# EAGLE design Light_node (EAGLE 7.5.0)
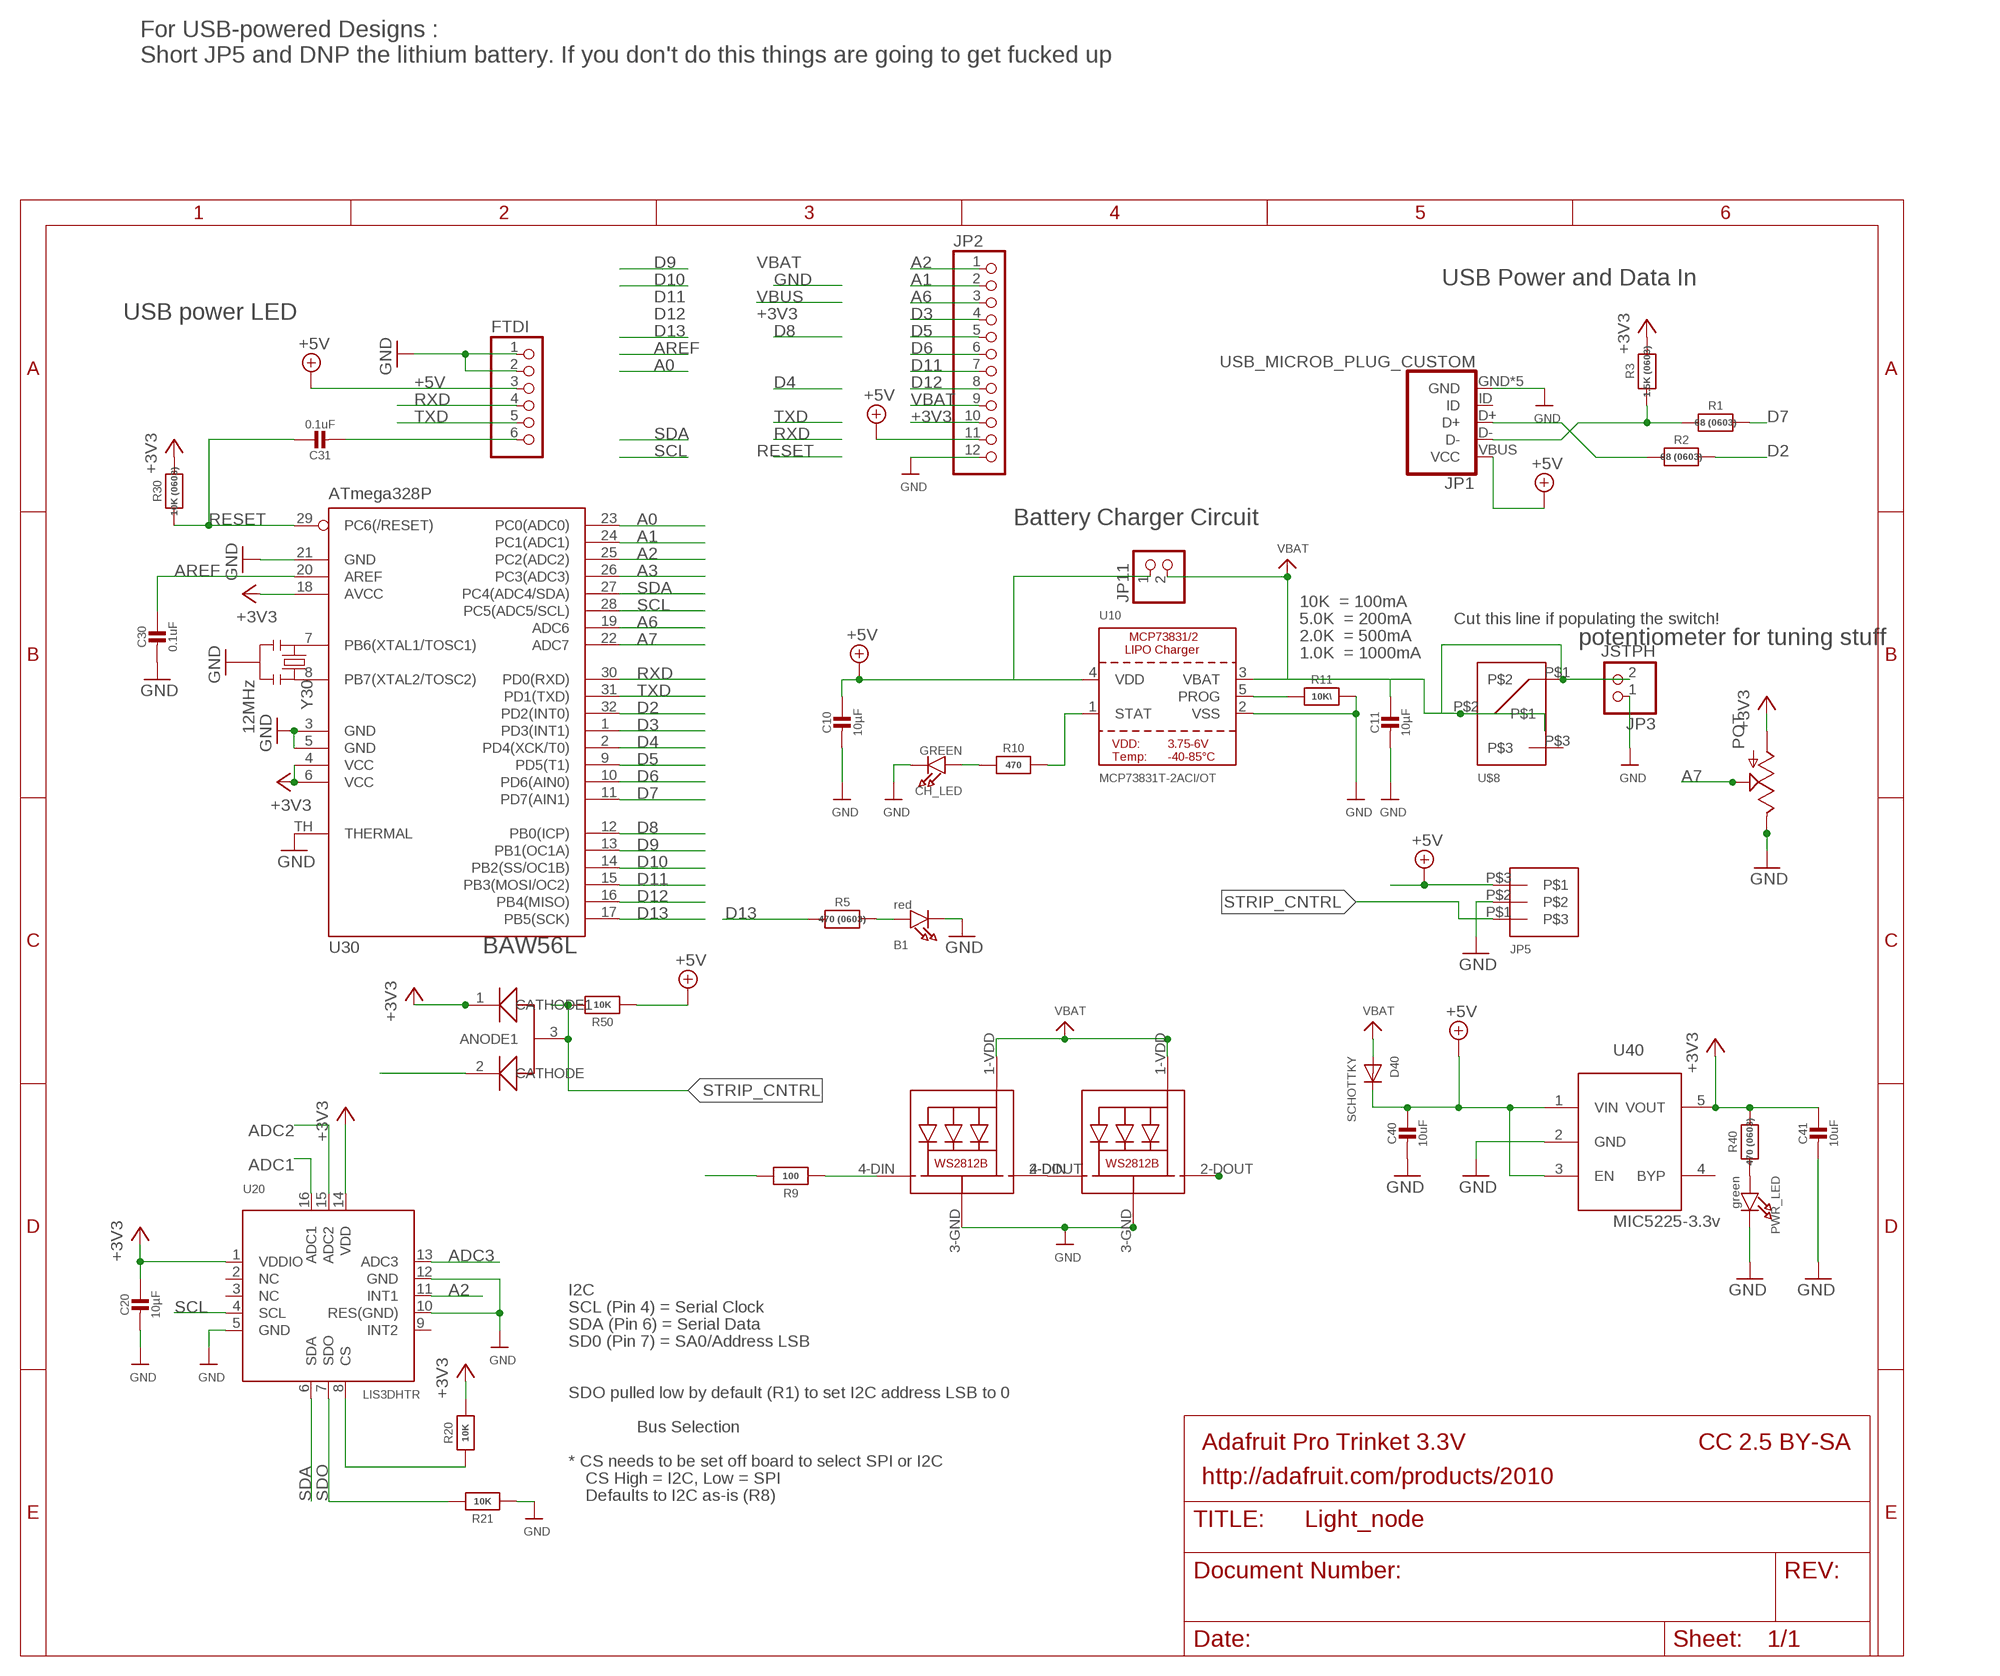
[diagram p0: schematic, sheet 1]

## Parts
B1  red  LED0805_NOOUTLINE  [CHIPLED_0805_NOOUTLINE]
C10  10µF  CAP_CERAMIC0805-NOOUTLINE  [0805-NO]
C11  10µF  CAP_CERAMIC0805-NOOUTLINE  [0805-NO]
C20  10µF  CAP_CERAMIC0805-NOOUTLINE  [0805-NO]
C30  0.1uF  CAP_CERAMIC_0805MP  [_0805MP]
C31  0.1uF  CAP_CERAMIC0805-NOOUTLINE  [0805-NO]
C40  10uF  CAP_CERAMIC0805-NOOUTLINE  [0805-NO]
C41  10uF  CAP_CERAMIC0805-NOOUTLINE  [0805-NO]
CH_LED  GREEN  LED0805_NOOUTLINE  [CHIPLED_0805_NOOUTLINE]
D40  SCHOTTKY  DIODE_SOD-123FL  [SOD-123FL]
FTDI  PINHD-1X6CB  [1X06-CLEANBIG]
JP1  USB_MICROB_PLUG_CUSTOM  [USB-MICROB]
JP2  PINHD-1X12-CB  [1X12-CB]
JP3  JSTPH  JST_2PIN  [JSTPH2]
JP5  M03  [M03_25MM]
JP11  HEADER-1X2ROUND  [1X02_ROUND]
POT  POT  [3306P_POT]
PWR_LED  green  LED0805_NOOUTLINE  [CHIPLED_0805_NOOUTLINE]
R1  68 (0603)  RESISTOR_0603_NOOUT  [0603-NO]
R2  68 (0603)  RESISTOR_0603_NOOUT  [0603-NO]
R3  1.5K (0603)  RESISTOR_0603_NOOUT  [0603-NO]
R5  470 (0603)  RESISTOR_0603_NOOUT  [0603-NO]
R9  100  RESISTOR_0603_NOOUT  [0603-NO]
R10  470  RESISTOR0805_NOOUTLINE  [0805-NO]
R11  10K\  RESISTOR0805_NOOUTLINE  [0805-NO]
R20  10K  RESISTOR0805_NOOUTLINE  [0805-NO]
R21  10K  RESISTOR0805_NOOUTLINE  [0805-NO]
R30  10K (0603)  RESISTOR0805_NOOUTLINE  [0805-NO]
R40  470 (0603)  RESISTOR_0603_NOOUT  [0603-NO]
R50  10K  RESISTOR_0603_NOOUT  [0603-NO]
RGB1  WS2812B5050  [WS2812B]
RGB2  WS2812B5050  [WS2812B]
U10  MCP73831T-2ACI/OT  MCP73831/2  [SOT23-5]
U20  LIS3DHTR  ACCEL_LIS3DHTR  [LGA16_3X3MM]
U30  ATmega328P  MEGA8-MI  [MLF32-TH]
U40  MIC5225-3.3v  LP298XS  [SOT23-5L]
U50  COMMON_ANODE_DIODE  [SOT23]
U$8  SPDT_NO_GNDSMT  [JS102011SAQN]
Y30  12MHz  RESONATORSMD  [RESONATOR-SMD]

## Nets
+3V3 [power]: C20.1 C41.1 JP2.10 POT.P$1(A) R3.2 R20.2 R30.2 R40.2 U20.1(VDDIO) U20.14(VDD) U30.4(VCC) U30.6(VCC) U30.18(AVCC) U40.5(VOUT) U50.1(CATHODE1)
+5V: C10.1 C40.1 D40.C FTDI.3 JP1.VBUS(VCC) JP2.11 JP5.P$3 JP11.1 R50.1 U10.4(VDD) U40.1(VIN) U40.3(EN)
A0: U30.23(PC0(ADC0))
A1: JP2.2 U30.24(PC1(ADC1))
A2: JP2.1 U20.11(INT1) U30.25(PC2(ADC2))
A3: U30.26(PC3(ADC3))
A6: JP2.3 U30.19(ADC6)
A7: POT.P$3(S) U30.22(ADC7)
ADC1: U20.16(ADC1)
ADC2: U20.15(ADC2)
ADC3: U20.13(ADC3)
AREF: C30.1 U30.20(AREF)
CS: R20.1 U20.8(CS)
D2: R2.2 U30.32(PD2(INT0))
D3: JP2.4 U30.1(PD3(INT1))
D4: U30.2(PD4(XCK/T0)) U50.2(CATHODE)
D5: JP2.5 U30.9(PD5(T1))
D6: JP2.6 U30.10(PD6(AIN0))
D7: R1.2 U30.11(PD7(AIN1))
D8: U30.12(PB0(ICP))
D9: U30.13(PB1(OC1A))
D10: R9.2 U30.14(PB2(SS/OC1B))
D11: JP2.7 U30.15(PB3(MOSI/OC2))
D12: JP2.8 U30.16(PB4(MISO))
D13: R5.2 U30.17(PB5(SCK))
D+: JP1.D+ R2.1
D-: JP1.D- R1.1 R3.1
DTR/RTS: C31.2 FTDI.6
GND [power]: B1.C C10.2 C11.2 C20.2 C30.2 C40.2 C41.2 CH_LED.C FTDI.1 FTDI.2 JP1.GND JP1.P$1(GND) JP1.P$2(GND) JP1.P$3(GND) JP1.P$4(GND) JP2.12 JP3.1 JP5.P$2 POT.P$2(E) PWR_LED.C R11.2 R21.1 RGB1.3-GND(GND) RGB2.3-GND(GND) U10.2(VSS) U20.5(GND) U20.10(RES(GND)) U20.12(GND) U30.3(GND) U30.5(GND) U30.21(GND) U30.TH(THERMAL) U40.2(GND) Y30.2
LED_CNTRL: R9.1 RGB1.4-DIN(DI)
N$1: B1.A R5.1
N$2: U30.8(PB7(XTAL2/TOSC2)) Y30.3
N$3: U30.7(PB6(XTAL1/TOSC1)) Y30.1
N$4: RGB1.2-DOUT(DO) RGB2.4-DIN(DI)
N$5: R10.2 U10.1(STAT)
N$6: PWR_LED.A R40.1
N$8: R11.1 U10.5(PROG)
N$9: CH_LED.A R10.1
N$15: RGB2.2-DOUT(DO)
RESET: C31.1 R30.1 U30.29(PC6(/RESET))
RXD: FTDI.4 U30.30(PD0(RXD))
SCL: U20.4(SCL) U30.28(PC5(ADC5/SCL))
SDA: U20.6(SDA) U30.27(PC4(ADC4/SDA))
SDO: R21.2 U20.7(SDO)
STRIP_CNTRL: JP5.P$1 R50.2 U50.3(ANODE1)
TXD: FTDI.5 U30.31(PD1(TXD))
VBAT [power]: C11.1 D40.A JP2.9 JP3.2 JP11.2 RGB1.1-VDD(VDD) RGB2.1-VDD(VDD) U10.3(VBAT) U$8.P$1 U$8.P$2
Unconnected: JP1.ID U20.2(NC) U20.3(NC) U20.9(INT2) U40.4(BYP) U$8.P$3

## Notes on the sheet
- For USB-powered Designs : 
  Short JP5 and DNP the lithium battery. If you don't do this things are going to get fucked up
- USB Power and Data In
- USB power LED
- Battery Charger Circuit
- 10K  = 100mA
- 5.0K  = 200mA | Cut this line if populating the switch!
- 2.0K  = 500mA | potentiometer for tuning stuff
- 1.0K  = 1000mA
- BAW56L
- I2C
- SCL (Pin 4) = Serial Clock
- SDA (Pin 6) = Serial Data
- SD0 (Pin 7) = SA0/Address LSB
- SDO pulled low by default (R1) to set I2C address LSB to 0
- Bus Selection
- Adafruit Pro Trinket 3.3V | CC 2.5 BY-SA
- * CS needs to be set off board to select SPI or I2C
- CS High = I2C, Low = SPI | http://adafruit.com/products/2010
- Defaults to I2C as-is (R8)

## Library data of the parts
B1 CH_LED PWR_LED = microbuilder:LED: LED
C10 C11 C20 C30 C31 C40 C41 = microbuilder:CAP_CERAMIC: Ceramic Capacitors
D40 = adafruit:DIODE: Diode
FTDI = adafruit:PINHD-1X6: PIN HEADER
JP1 = 0_AlpineLabs:USB_MICROB_PLUG: USB Micro-B Plug Comes in a variety of packages. Check out Hirose's ZX-x0 line: http://www.hirose.co.jp/cataloge_hp/e24200011.pdf
JP2 = adafruit:PINHD-1X12: PIN HEADER
JP3 = microbuilder:JST_2PIN: JST 2-Pin Right-Angle Connector
JP5 = 0_Shibbs1:M03
JP11 = microbuilder:HEADER-1X2: PIN HEADER
POT = 0_Shibbs1:POT
R1-R3 R5 R9-R11 R20 R21 R30 R40 R50 = microbuilder:RESISTOR: Resistors
RGB1 RGB2 = microbuilder:WS2812B5050
U10 = microbuilder:MCP73831/2: MCP73831/2 LIPO Charger VDD: 3.75 - 6V Temp -40 - 85°C Programmable Charge Rate: 15-500mA NOTE: STAT is a tri-state logic output on the MCP73831 and an open-drain output on the MCP73832. SOT23-5 with 4.2V output and tri-state logic on STAT = MCP73831T-2ACI/OT
U20 = microbuilder:ACCEL_LIS3DHTR: LIS3DHTR 3-Axis Accelerometer with I2C/SPI Interface VDD: 1.71-3.6V VDDIO: 1.71-VDD+0.1V Scale: +/-2g, 4g, 8g, 16g with 16--bit data output Temp:: -40°C - 85°C Mouser: 511-LIS3DHTR Digikey: 497-10613-1-ND
U30 = microbuilder:MEGA8-MI: MICROCONTROLLER 8 Kbytes FLASH, 1 kbytes SRAM, 512 bytes EEPROM, USART, 6-channel 10 bit ADC, 2-channel 8 bit ADC Pin compatible with Atmega48, ATMega88, ATMega168 Source: avr.lbr; MPN: ATMEGA88PA-MU; OC_FARNELL: 1715491; OC_NEWARK: 15R0272
U40 = adafruit:LP298X
U50 = 0_AlpineLabs:COMMON_ANODE_DIODE
U$8 = 0_Shibbs1:SPDT_NO_GND
Y30 = SparkFun:RESONATOR: Resonator Small SMD resonator. This is the itty bitty 10/20MHz resonators with built in caps. CSTCE10M0G55 and CSTCE20M0V53. Footprint has been reviewed closely but hasn't been tested yet.

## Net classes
1 power: width 0.305 mm

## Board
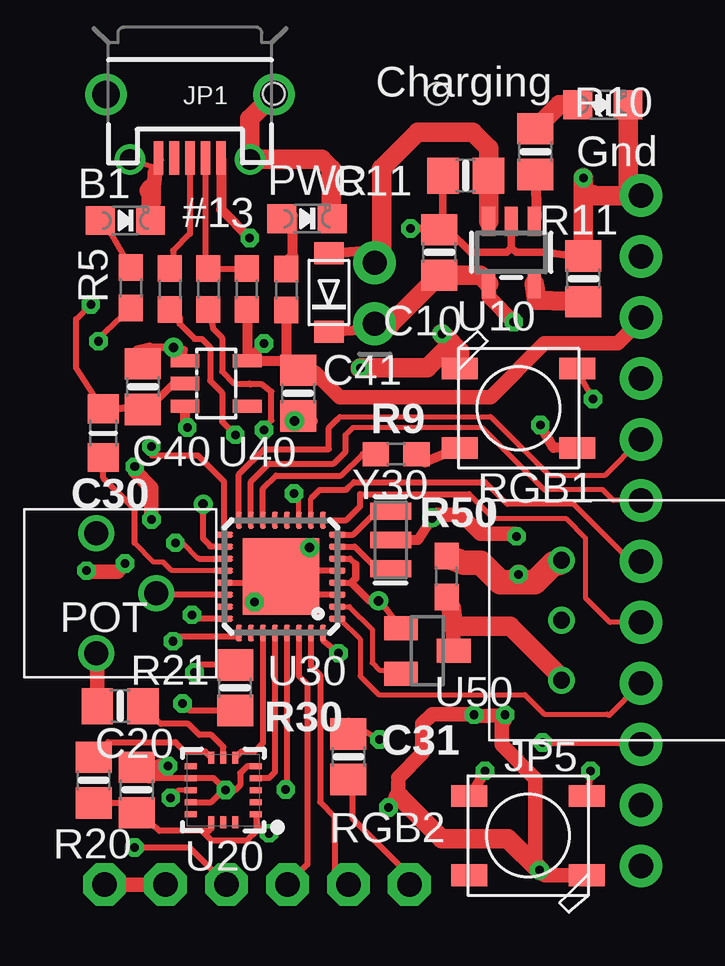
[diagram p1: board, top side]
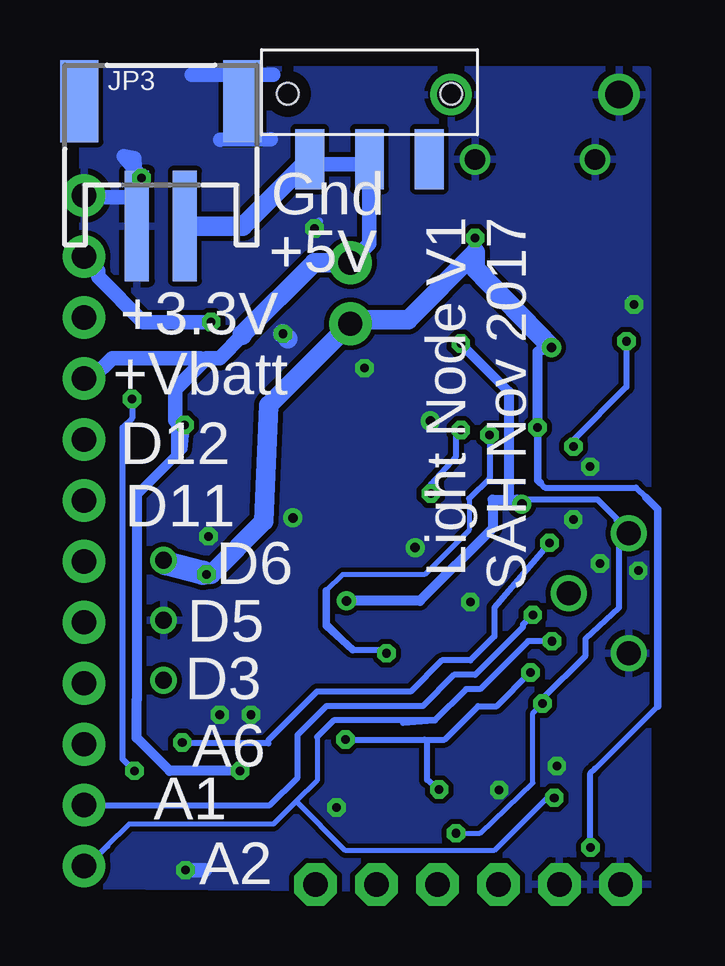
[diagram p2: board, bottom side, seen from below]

No outline drawn. Coordinates in mm, seen from the top.
Copper layers (1*16): Top 0.0178mm / dielectric 59mil / Bottom 0.0178mm
Design rules "SSC-EAGLE-2Lyr_v1.0.0.3 *": minimum track width 6mil, minimum drill 14mil, track to track 8mil, track to pad 8mil, pad to pad 8mil, via to via 8mil, smd to smd 6mil, copper to edge 20mil, drill to drill 16mil, minimum pad ring 8mil, minimum via ring 8mil, stop-mask expansion 3mil, vias tented up to drill 0mil, thermal gap 10mil

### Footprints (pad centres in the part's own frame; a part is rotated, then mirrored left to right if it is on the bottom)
CHIPLED_0805_NOOUTLINE = smd 1.2 x 1.2: A 0,-1.05; C 0,1.05
0805-NO = smd 1.3 x 1.5: 1 -0.95,0; 2 0.95,0
_0805MP = smd 1.2 x 1.3: 1 -1.016,0; 2 1.016,0
SOD-123FL = smd 0.91 x 1.22: A 1.637,0; C -1.637,0
1X06-CLEANBIG = drill 1.016 pad 1.778 octagon: 1 -6.35,0; 2 -3.81,0; 3 -1.27,0; 4 1.27,0; 5 3.81,0; 6 6.35,0
USB-MICROB = smd 0.4 x 1.4: D+ 0,2.65; D- -0.65,2.65; GND 1.3,2.65; ID 0.65,2.65; VBUS -1.3,2.65 | drill 1.15 pad 1.201: P$1 -3.5,0; P$2 3.5,0 | drill 0.85 pad 0.914: P$3 -2.5,2.7; P$4 2.5,2.7
1X12-CB = drill 1.016 pad 1.778: 1 -13.97,0; 2 -11.43,0; 3 -8.89,0; 4 -6.35,0; 5 -3.81,0; 6 -1.27,0; 7 1.27,0; 8 3.81,0; 9 6.35,0; 10 8.89,0; 11 11.43,0; 12 13.97,0
JSTPH2 = smd 1 x 4.6: 1 -1,-3.7; 2 1,-3.7 | smd 1.6 x 3.4: NC1 -3.4,1.5; NC2 3.4,1.5
M03_25MM = drill 0.7: P$1 0,-2.5; P$2 0,0; P$3 0,2.5
1X02_ROUND = drill 1 pad 1.778: 1 -1.27,0; 2 1.27,0
3306P_POT = drill 1: P$1 -2.5,0; P$2 2.5,0; P$3 0,2.5
0603-NO = smd 1.1 x 1: 1 -0.85,0; 2 0.85,0
WS2812B = smd 1.5 x 0.9: 1-VDD 2.45,-1.65; 2-DOUT 2.45,1.65; 3-GND -2.45,1.65; 4-DIN -2.45,-1.65
SOT23-5 = smd 0.55 x 1.2: 1 -0.95,-1.3; 2 0,-1.3; 3 0.95,-1.3; 4 0.95,1.3; 5 -0.95,1.3
LGA16_3X3MM = smd 0.5 x 0.25: 1 -1.35,1; 2 -1.35,0.5; 3 -1.35,0; 4 -1.35,-0.5; 5 -1.35,-1; 9 1.35,-1; 10 1.35,-0.5; 11 1.35,0; 12 1.35,0.5; 13 1.35,1 | smd 0.25 x 0.5: 6 -0.5,-1.35; 7 0,-1.35; 8 0.5,-1.35; 14 0.5,1.35; 15 0,1.35; 16 -0.5,1.35
MLF32-TH = smd 0.7 x 0.25: 1 -2.35,1.75; 2 -2.35,1.25; 3 -2.35,0.75; 4 -2.35,0.25; 5 -2.35,-0.25; 6 -2.35,-0.75; 7 -2.35,-1.25; 8 -2.35,-1.75; 17 2.35,-1.75; 18 2.35,-1.25; 19 2.35,-0.75; 20 2.35,-0.25; 21 2.35,0.25; 22 2.35,0.75; 23 2.35,1.25; 24 2.35,1.75 | smd 0.25 x 0.7: 9 -1.75,-2.35; 10 -1.25,-2.35; 11 -0.75,-2.35; 12 -0.25,-2.35; 13 0.25,-2.35; 14 0.75,-2.35; 15 1.25,-2.35; 16 1.75,-2.35; 25 1.75,2.35; 26 1.25,2.35; 27 0.75,2.35; 28 0.25,2.35; 29 -0.25,2.35; 30 -0.75,2.35; 31 -1.25,2.35; 32 -1.75,2.35 | smd 3.2 x 3.2: TH 0,0
SOT23-5L = smd 0.55 x 1.2: 1 -0.95,-1.3; 2 0,-1.3; 3 0.95,-1.3; 4 0.95,1.3; 5 -0.95,1.3
SOT23 = smd 1 x 1.4: 1 -0.95,-1.1; 2 0.95,-1.1; 3 0,1.1
JS102011SAQN = smd 1.2 x 2.5: P$1 2.489,2.794; P$2 0,2.794; P$3 -2.489,2.794 | hole 0.889: 3.404,0.064; -3.404,0.064
RESONATOR-SMD = smd 0.7 x 1.7: 1 -1.2,0; 2 0,0; 3 1.2,0

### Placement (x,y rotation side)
B1  3.01,29.15 270 top
C10  16.09,27.82 90 top
C11  17.19,31.02 180 top
C20  3.49,5.43 90 top
C30  2.09,20.3 90 top
C31  12.3,6.81 270 top
C40  3.75,22.23 270 top
C41  10.22,21.96 270 top
CH_LED  22.91,33.98 270 top
D40  11.49,26.15 90 top
FTDI  8.49,1.49 0 top
JP1  5.7,34.4 180 top
JP2  24.49,16.22 90 top
JP3  21.29,32.62 0 bottom
JP5  21.18,12.5 0 top
JP11  13.39,26.12 90 top
POT  1.79,13.62 270 top
PWR_LED  10.58,29.23 270 top
R1  6.47,26.3 270 top
R2  4.87,26.3 270 top
R3  8.06,26.3 270 top
R5  3.24,26.35 270 top
R9  14.29,19.42 180 top
R10  20.09,32.02 270 top
R11  22.09,26.72 90 top
R20  1.69,5.84 270 top
R21  2.79,8.92 0 top
R30  7.58,9.68 270 top
R40  9.72,26.27 270 top
R50  16.39,14.32 270 top
RGB1  19.39,21.33 0 top
RGB2  19.79,3.52 180 top
U10  19.09,27.82 180 top
U20  7.09,5.42 180 top
U30  9.49,14.32 180 top
U40  6.79,22.36 270 top
U50  15.59,11.22 270 top
U$8  12.6,34.5 180 bottom
Y30  14.07,15.84 90 top

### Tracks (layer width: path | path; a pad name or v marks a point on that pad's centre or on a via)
+3V3  (via drill 0.36, 0.39)
  Top 0.203: U20.1 8.54,3.87 v8.99,3.62 | U20.14 6.59,3.82
  Top 0.254: U30.18 6.55,15.57 6.55,15.6 6.25,15.9 v6.25,17.33 | U30.6 12.36,15.07 12.61,14.83 | U30.4 12.41,14.07 12.41,14.06 | R30.2 5.68,8.73 v5.39,9.02 | U50.1 13.89,12.97 v13.56,13.3 | 6.59,3.82 6.49,3.72 6.19,3.72 | 6.19,3.72 4.44,3.72 C20.1 3.08,4.88 R20.2 | 6.19,3.72 6.59,3.32 8.1,3.32 8.48,3.71 8.48,4.38 U20.1
  Top 0.305: 12.61,14.83 12.61,14.26 12.41,14.06 13.18,13.3 v13.56,13.3
  Top 0.406: 8.19,23.41 U40.5 | U40.5 9.69,23.31 | 9.69,23.31 C41.1 | R3.2 8.09,25.41 U40.5 | R40.2 9.72,23.33 9.69,23.31 | v8.79,24.02 8.79,24.01 U40.5
  Top 0.61: JP2.10 24.49,25 23.52,24.03 20.47,24.03 18.24,21.79 11.94,21.79 10.92,22.81 10.31,22.81 C41.1
  Bottom 0.203: v8.99,3.62 7.99,3.62 5.79,5.72 5.79,8.62 v5.39,9.02
  Bottom 0.254: v5.39,9.02 5.39,9.22 3.59,11.02 3.59,11.72 2.19,13.02 2.19,15.62 POT.P$1 2.29,16.62 2.29,16.72 3.09,17.52 6.06,17.52 v6.25,17.33 | 6.44,17.53 6.68,17.53 6.79,17.64
  Bottom 0.406: v8.79,24.02 6.79,22.02 6.79,17.64 | v6.25,17.33 6.44,17.53 7.47,17.53 7.47,16.33 10.5,13.3 v13.55,13.3 v13.56,13.3
+5V  (via drill 0.36, 0.39)
  Top 0.254: U40.1 5.49,23.79 v5.02,23.86 | v3.39,3.02 5.69,3.02 FTDI.3
  Top 0.305: C40.1 3.49,23.43 | 4.01,23.86 v5.02,23.86
  Top 0.406: 3.49,23.43 3.49,23.74 4.01,23.86 | D40.C 13.15,24.61 JP11.1 | U40.3 5.49,20.62 v5.59,20.52 | JP1.VBUS 7,29.62 v8.19,28.42
  Top 0.61: U10.4 18.14,25.97 v19.19,24.92
  Top 0.813: JP11.1 14.07,24.85 C10.1 17.79,26.87 U10.4 | 19.42,13.98 v19.39,14.41 | 21.06,14.87 JP5.P$3
  Top 1.016: 21.06,14.87 20.86,14.87 20.07,14.07 18.64,14.07 17.83,14.88 17.11,14.88 R50.1
  Bottom 0.203: 3.2,6.32 0.59,8.92
  Bottom 0.254: 5.02,24.09 v5.02,23.86 | 5.49,18.22 5.29,18.02 1.5,18.02 1.09,17.61 | v3.39,3.02 3.39,6.12 3.2,6.32
  Bottom 0.305: v5.59,20.52 5.59,18.32 5.49,18.22 | 1.09,17.61 0.59,17.11 0.59,8.92
  Bottom 0.406: v8.19,28.42 8.19,27.82 | 13.22,25.02 JP11.1 | v5.59,20.52 5.59,23.68 v5.02,23.86
  Bottom 0.61: 24.46,27.69 JP2.11 23.9,27.06 23.9,26.8 22.02,24.92 v19.19,24.92
  Bottom 0.813: JP11.1 16.79,21.45 17,16.61 19.2,14.41 v19.39,14.41 19.54,14.47 | 13.22,25.02 10.99,25.02 8.19,27.82 8.19,27.14 v5.02,23.86
  Bottom 1.016: 19.54,14.47 21.06,14.87 JP5.P$3
A1  (via drill 0.36)
  Top 0.254: U30.24 5.95,12.57 v5.79,12.72
  Bottom 0.254: v5.79,12.72 6.19,12.32 6.19,12.22 8.19,10.22 9.08,10.22 10.38,8.92 14.39,8.92 15.59,7.72 15.59,5.94 16.75,4.79 JP2.2
A2  (via drill 0.36)
  Top 0.203: U20.11 5.22,5.42 v4.9,5.1
  Top 0.254: U30.25 7.74,11.81 5.18,11.81 v4.99,11.62
  Bottom 0.203: 14.78,7.63 14.78,5.82 15.65,4.95 | 15.65,4.95 16.6,4 22.62,4 23.52,3.1 | v4.9,5.1 5.2,5.1 7.4,2.9 13.6,2.9 15.65,4.95
  Bottom 0.254: v4.99,11.62 5.99,11.62 7.99,9.62 8.57,9.62 9.87,8.32 | 11.19,8.22 9.87,8.32 | 9.87,8.32 14.09,8.32 14.78,7.63 | JP2.1 24.37,2.25 23.52,3.1
A6  (via drill 0.36)
  Top 0.203: U30.19 6.05,15.07 5.39,15.72 v5.09,15.72
  Top 0.254: 6.08,15.07 U30.19 | v20.4,7.4 24.43,7.4 JP2.3
  Bottom 0.254: v5.09,15.72 7.39,13.02 7.39,11.82 8.39,10.82 9.58,10.82 10.88,9.52 14.79,9.52 16.81,7.5 16.81,7.37 20.07,7.37 v20.4,7.4
A7
  Top 0.254: U30.22 4.35,13.57 POT.P$3
AREF
  Top 0.203: U30.20 4.95,14.57 4.59,14.92 4.19,14.92 3.39,15.72
  Top 0.254: C30.1 2.09,19.08 2.09,18.42 3.39,17.12 3.39,15.72
CS
  Top 0.254: 6.59,6.82 U20.8 6.34,7.02 5.49,7.02 5.09,7.42 2.29,7.42 2.29,7.22 2.19,7.12 2.19,6.47 R20.1
D2  (via drill 0.36)
  Top 0.254: R2.2 5.27,25.15 5.27,24.85 5.89,24.22 6.2,24.22 6.54,23.88 6.54,22.48 7.05,21.98 7.05,20.77 v7.59,20.22 | U30.32 11.24,11.67 v11.89,11.12
  Bottom 0.203: 8.45,17.57 8.45,16.25 10.3,14.4 13.72,14.4 14.39,13.72
  Bottom 0.254: 14.32,12.29 13.3,11.27 12.04,11.27 v11.89,11.12 | v7.59,20.22 7.59,18.42 8.45,17.57
  Bottom 0.305: 14.39,13.72 14.39,12.26 13.3,11.27
D3
  Top 0.203: U30.1 11.95,12.57 12.79,11.72 12.79,10.17 13.56,9.4 19.66,9.4 20.47,8.59 23.08,8.59 23.14,8.52 JP2.4
D4
  Top 0.203: U30.2 12.35,13.07 13.29,12.12 13.29,10.72 13.59,10.42 14.44,10.42 U50.2
D5
  Top 0.203: JP2.5 23.2,12.41 22.19,13.42 22.19,15.92 21.39,16.72 18.36,16.72 17.34,17.75
  Top 0.254: U30.9 12.22,16.67 12.8,17.24 12.8,17.75 17.34,17.75
D6
  Top 0.203: JP2.6 24.06,14.95 21.69,17.32 18.93,17.32 18,18.26 | U30.10 10.74,17.57 10.79,17.62
  Top 0.254: 18,18.26 12.54,18.26 12.29,18 12.27,18 12.19,17.92 11.09,17.92 10.79,17.62
D7  (via drill 0.36)
  Top 0.203: U30.11 10.24,17.57 v10.04,17.77
  Top 0.254: R1.2 6.67,24.64 7.05,24.26 7.05,22.87 7.56,22.36 8.19,22.36 8.23,22.32 8.69,22.32 9.09,22.02 9.09,20.82 v8.79,20.42
  Bottom 0.254: v10.04,17.77 10.04,18.17 8.99,19.32 8.99,20.42 v8.79,20.42
D10
  Top 0.254: U30.14 8.74,17.97 9.29,18.52 11.99,18.52 12.89,19.42 R9.2
D11
  Top 0.203: JP2.7 23.35,17.49 22.91,17.93 20.47,17.93 17.88,20.52 12.49,20.52 12.19,20.22
  Top 0.254: U30.15 8.24,18.27 8.99,19.02 11.69,19.02 12.19,19.52 12.19,20.22
D12
  Top 0.203: 11.84,20.87 11.95,20.98 18.24,20.98 20.67,18.54 23,18.54 JP2.8
  Top 0.254: U30.16 7.74,18.57 8.79,19.62 11.49,19.62 11.49,20.52 11.84,20.87
D13  (via drill 0.36)
  Top 0.254: U30.17 7.14,16.29 7.13,16.29 7.13,18.27 6.04,19.36 4.13,19.36 v4.09,19.73 | R5.2 1.84,24.18 v1.89,24.12
  Bottom 0.254: v1.89,24.12 1.89,22.22 4.09,20.02 v4.09,19.73
D+
  Top 0.254: JP1.D+ 5.7,28.6 5,27.9 5,27.28 R2.1
D-
  Top 0.254: R3.1 R1.1 6.35,27.26 JP1.D-
DTR/RTS
  Top 0.254: FTDI.6 14.84,1.87 12.49,4.22 12.49,5.67 C31.2
GND  (via drill 0.36, 0.39)
  Top 0.203: 4.14,5.92 4.29,5.92 v4.79,6.42 | JP1.P$4 4.3,31.34 4.16,31.2
  Top 0.254: U30.5 9.74,14.57 | U30.3 10.24,13.57 | U30.21 9.24,14.07 | U20.12 6.59,4.92 7.09,5.42 7.09,5.52 | 7.09,5.52 6.69,5.92 U20.10 4.14,5.92 C20.2 | U20.5 8.09,6.42 7.79,6.12 7.79,5.62 7.59,5.42 v7.19,5.42 7.09,5.52 | C30.2 1.86,21.61 0.96,23.01 0.96,25.05 v1.57,25.65
  Top 0.305: 9.24,14.07 v10.69,15.52 | 9.74,14.57 v10.69,15.52 | 10.24,13.57 v10.69,15.52 | C30.2 3.69,21.34 C40.2 4.06,21.6 4.25,21.6 5.02,22.36 U40.2 | U10.2 19.09,28.02 | 19.09,28.02 19.29,27.82 20.49,27.82 21.29,27.72 21.84,27.82 | C10.2 16.44,28.77 17.39,27.82 18.89,27.82 19.09,28.02 | C11.2 16.24,28.92 C10.2 | C10.2 16.09,28.82 v14.89,28.82
  Top 0.406: Y30.2 15.21,15.84 v15.79,16.76 | B1.C 4.16,31.2 | C41.2 10.82,20.8 v10.06,20.8 | JP1.GND 4.3,30.7 4,30.4
  Top 0.61: R21.1 1.84,11.07 POT.P$2 | RGB2.3-GND 20.48,1.87 v20.27,2.08 | v3,14.86 2.93,14.76 2.69,14.52 1.53,14.52 v1.4,14.56 | 14.38,5.94 15.39,6.96 15.39,8.18 15.8,8.59 17.51,8.59 v17.54,8.56 17.59,8.5 arc45 17.6,8.5 18.87,8.53 | 14.38,5.74 14.38,5.13 14.04,4.79 v13.98,4.7 | v19.3,15.99 19.3,16.05 19.25,16.1 17.8,16.1 17,16.9 16,16.9 15.8,16.7 | 3.39,18.82 3.39,18.72 4.09,18.02 4.09,16.71 | 4.09,16.71 4.09,16.62 | v4.1,16.7 4.09,16.71 | 4.62,1.47 2.16,1.47 FTDI.1 | v4.79,6.42 4.42,6.42 4,6 | PWR_LED.C 11.63,30.57 | 22.11,30.23 22.5,30.23 24,30.23 24.21,30.23 | 20.2,2.2 20.19,2.21 arc-45 20.1,2.43 20.1,5.9 18.7,7.3 18.7,8.09 arc-45 18.79,8.31 v18.84,8.56
  Top 0.813: RGB1.3-GND 16.94,23.7 16.61,24.03 | 16.61,24.03 v16.2,24.43 | v12.81,23 12.82,23.01 15.59,23.01 16.61,24.03 | 14.38,5.13 14.47,5.13 16.2,3.4 18.95,3.4 v20.27,2.08 | 4,30.4 4.1,30.49 B1.C | v22.09,30.93 R11.2 | JP2.12 22.54,30.19 22.5,30.23 | CH_LED.C 23.96,30.27 24,30.23 | PWR_LED.C 11.6,29.26 11.6,31.3 11.2,31.7 JP1.P$3 8.2,33.4 JP1.P$1
  Top 1.016: 9.74,14.57 U30.TH
  Bottom 0.203: 4.79,2.05 4.62,1.88
  Bottom 0.254: v1.57,25.65 1.78,25.86
  Bottom 0.305: v14.89,28.82 14.99,28.82 14.69,29.12
  Bottom 0.61: v20.27,2.08 19.45,2.08 | v22.09,30.93 22.84,31.82 22.41,31.75 22.31,30.13 24.41,30.13 | 16.61,35.23 20.01,35.23 | 16.71,32.53 18.81,32.53
  Bottom 0.813: v16.2,24.43 16,24.23
  other vias: 8.4,13.26 3.4,18.9
  pour Bottom: 1.01,35.43 1.01,1.24 24.55,1.44 24.55,35.43
LED_CNTRL
  Top 0.406: RGB1.4-DIN 15.49,19.07 R9.1
N$1
  Top 0.254: R5.1 1.84,29.63 B1.A
N$2
  Top 0.254: U30.8 12.51,16.07 13.43,16.99 14.01,16.99 Y30.3
N$3
  Top 0.254: U30.7 12.56,15.57 13.49,14.64 Y30.1
N$4  (via drill 0.36)
  Top 0.254: RGB1.2-DOUT 21.94,22.67 v22.49,21.72 | v22.39,6.22 22.39,6.12 RGB2.4-DIN
  Bottom 0.254: v22.49,21.72 22.49,20.92 22.89,20.52 22.89,6.72 v22.39,6.22
N$5
  Top 0.406: R10.2 20.14,29.22 U10.1
N$6
  Top 0.406: R40.1 9.72,27.45 9.99,27.72 9.99,29.37 PWR_LED.A
N$8
  Top 0.813: U10.5 20.14,25.82 R11.1
N$9
  Top 0.813: CH_LED.A 21.1,33.98 R10.1
RESET  (via drill 0.36)
  Top 0.254: U30.29 9.74,5.19 v9.69,5.44 | R30.1 6.18,10.63 v5.89,10.32 | C31.1 12.3,8.31 v13.59,7.52
  Bottom 0.254: v9.69,5.44 10.19,5.85 10.19,7.41 10.31,7.52 | v13.59,7.52 10.31,7.52 | 10.31,7.52 9.47,7.52 8.07,8.92 7.29,8.92 v5.89,10.32
RXD
  Top 0.254: U30.30 10.24,10.17 10.59,9.82 10.59,2.32 FTDI.4
SCL
  Top 0.254: U30.28 9.24,6.17 8.99,5.92 U20.4
SDA
  Top 0.254: U30.27 8.74,7.37 8.39,7.02 7.84,7.02 U20.6
SDO
  Top 0.254: U20.7 7.09,7.22 6.59,7.72 6.09,7.72 5.64,8.18 4.49,8.18 R21.2
STRIP_CNTRL
  Top 0.406: R50.2 16.59,13.02
  Top 0.61: U50.3 16.69,11.42 16.59,13.02
  Top 0.813: JP5.P$1 21.3,10 19.05,12.24 16.67,12.24 16.59,13.02
TXD
  Top 0.254: 12.39,1.58 FTDI.5 11.73,2.06 11.73,4.32 11.12,4.93 11.12,10.21 10.74,10.59 U30.31
VBAT  (via drill 0.36)
  Top 0.406: D40.A 12.9,27.89 JP11.2 | RGB2.1-VDD 17.94,6.07 v17.99,6.22 | RGB1.1-VDD 20.85,19.68 v20.3,20.64
  Top 0.813: JP11.2 13.69,27.69 13.69,31.32 15.19,32.82 17.49,32.82 18.14,32.17 C11.1 U10.3
  Bottom 0.406: 20.69,20.82 20.67,20.8 20.67,19.34 | 20.67,19.34 22.29,17.72 22.29,9.19 22.3,9.18 22.3,7.6 20.92,6.22 v17.99,6.22 | v20.3,20.64 20.39,19.62 20.67,19.34
  Bottom 0.61: 13.49,27.49 JP11.2 12.6,28.19 12.6,31.5 | 20.69,20.82 20.69,22.12 19.53,23.29 | JP2.9 24.16,22.57 23.32,23.42 19.66,23.42 19.53,23.29 | 17.89,24.37 18.85,23.42 19.4,23.42 19.53,23.29 | U$8.P$2 12.6,31.5 | 12.6,31.5 15,31.5 arc-45 U$8.P$1
  Bottom 0.813: 12.89,27.39 13,27.79 JP11.2 14.9,27.4 17.89,24.41 17.89,24.37 | JP3.2 17.87,28.92 U$8.P$1

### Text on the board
tPlace: Charging | Gnd | PWR | #13
bPlace: USBtinyISP / or UNO FTDI / Bootloader
bNames: Light Node V1 / SAH Nov 2017 | Gnd | +5V | +3.3V | +Vbatt | D12 | D11 | D6 | D5 | D3 | A6 | A1 | A2

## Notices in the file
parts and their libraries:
microbuilder: This work is placed in the public domain, and may be freely used for commercial and non-commercial work with the following conditions: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
SparkFun: Licensing: CC v3.0 Share-Alike You are welcome to use this library for commercial purposes.
